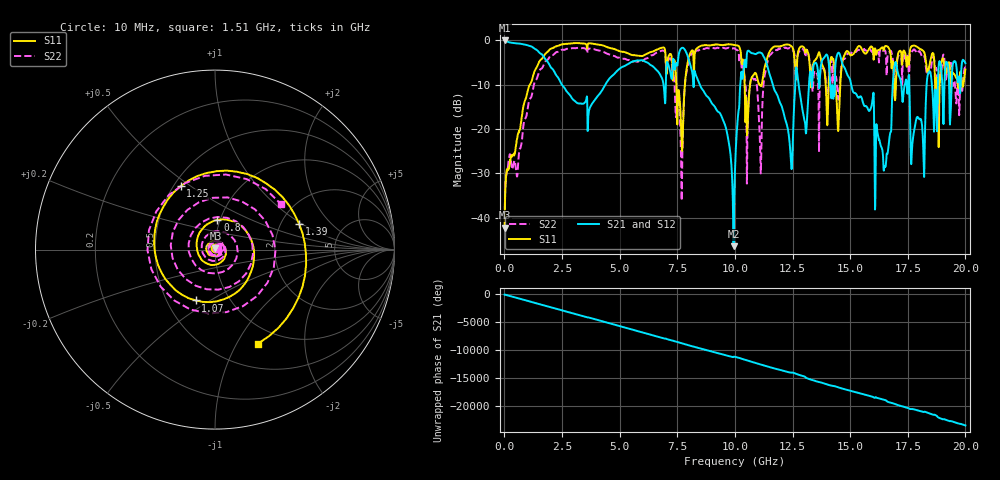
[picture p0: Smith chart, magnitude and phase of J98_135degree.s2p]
!Keysight Technologies,N5222A,MY51421036,A.10.65.16
!Date: Friday, March 31, 2023 15:16:48
!Correction: S11(Full 2 Port(1,2))
!S21(Full 2 Port(1,2))
!S12(Full 2 Port(1,2))
!S22(Full 2 Port(1,2))
!S2P File: Measurements: S11, S21, S12, S22:
# Hz S  dB  R 50
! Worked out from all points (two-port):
!   2000 points, 10 MHz to 20 GHz, reference 50 ohm
!   highest |S21| = -0.01 dB at 10 MHz (marker M1); lowest = -46.4 dB at 9.94 GHz (marker M2)
!   |S21| within 3 dB of the highest: start of sweep to 1.583 GHz; 7.571 GHz to 7.916 GHz (345 MHz wide, 4.46 % of centre)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
!   lowest |S11| = -42.2 dB at 10 MHz (marker M3), VSWR 1.02, Z = 50.2 + j0.744 ohm
!   |S11| at or under -10 dB: start of sweep to 1.108 GHz; 7.461 GHz to 7.83 GHz (368.9 MHz wide, 4.83 % of centre); 14.34 GHz to 14.57 GHz (233 MHz wide, 1.61 % of centre)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
!   |S22| runs from -37.9 to -1.6 dB; largest |S21 - S12| = 0.011
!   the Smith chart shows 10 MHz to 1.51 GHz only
!   S11 on the Smith chart (normalised r, x): 10 MHz: 1.00, +0.01; 800 MHz: 0.97, +0.33; 1.07 GHz: 0.69, -0.43; 1.25 GHz: 0.54, +0.46; 1.39 GHz: 2.50, +0.95; 1.51 GHz: 0.78, -1.23
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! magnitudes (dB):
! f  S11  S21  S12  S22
! 10 MHz  -42.2  0.0  0.0  -37.9
! 800 MHz  -15.6  -0.8  -0.8  -20.4
! 1.07 GHz  -10.4  -1.2  -1.2  -13.7
! 1.25 GHz  -7.9  -1.6  -1.6  -10.8
! 1.39 GHz  -6.2  -2.1  -2.1  -8.8
! 1.51 GHz  -4.8  -2.7  -2.7  -7.0
! 3.35 GHz  -0.7  -14.3  -14.3  -1.8
! 6.68 GHz  -1.9  -7.1  -7.1  -2.7
! 7.68 GHz  -21.4  -1.7  -1.7  -31.9
! 8.11 GHz  -2.4  -6.3  -6.2  -3.1
! 9.94 GHz  -1.0  -46.4  -46.4  -1.8
! 10.01 GHz  -1.1  -28.4  -28.3  -1.9
! 10.61 GHz  -12.7  -2.4  -2.4  -12.5
! 12.42 GHz  -1.1  -26.2  -26.2  -1.7
! 12.68 GHz  -6.5  -6.4  -6.4  -5.8
! 13.05 GHz  -2.6  -18.8  -18.8  -3.5
! 13.34 GHz  -7.8  -10.5  -10.5  -8.5
! 14.52 GHz  -15.8  -2.8  -2.8  -12.3
! 16.67 GHz  -1.7  -23.5  -23.6  -2.8
! 16.97 GHz  -12.2  -4.8  -4.8  -10.6
! 17.71 GHz  -1.2  -22.8  -22.7  -2.3
! 20 GHz  -6.5  -5.1  -5.1  -6.1
